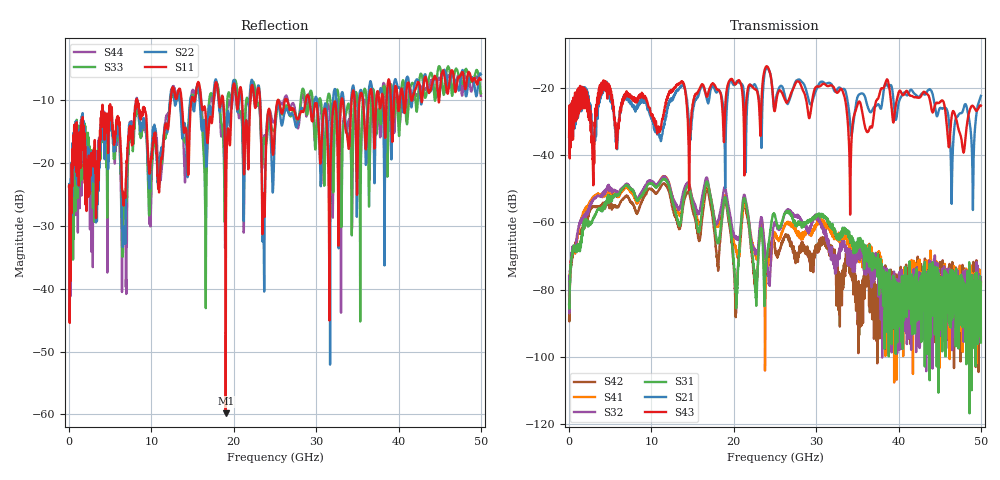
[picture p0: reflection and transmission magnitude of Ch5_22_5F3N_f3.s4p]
!Agilent Technologies,N5247A,US51170199,A.09.90.13
!Agilent N5247A: A.09.90.13
!Date: Wednesday, December 09, 2015 09:21:04
!Correction: S11(Full 4 Port(1,2,3,4))
!S12(Full 4 Port(1,2,3,4))
!S13(Full 4 Port(1,2,3,4))
!S14(Full 4 Port(1,2,3,4))
!S21(Full 4 Port(1,2,3,4))
!S22(Full 4 Port(1,2,3,4))
!S23(Full 4 Port(1,2,3,4))
!S24(Full 4 Port(1,2,3,4))
!S31(Full 4 Port(1,2,3,4))
!S32(Full 4 Port(1,2,3,4))
!S33(Full 4 Port(1,2,3,4))
!S34(Full 4 Port(1,2,3,4))
!S41(Full 4 Port(1,2,3,4))
!S42(Full 4 Port(1,2,3,4))
!S43(Full 4 Port(1,2,3,4))
!S44(Full 4 Port(1,2,3,4))
!S4P File: Measurements: <S11,S12,S13,S14>,
!<S21,S22,S23,S24>,
!<S31,S32,S33,S34>,
!<S41,S42,S43,S44>:
# Hz S  dB  R 50
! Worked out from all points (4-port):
!   3201 points, 10 MHz to 50 GHz, reference 50 ohm
!   strongest paths, dB at 10 MHz, 12.51 GHz, 25 GHz, 37.5 GHz, 50 GHz:
!     S43: -34.5, -21.0, -26.5, -23.2, -25.2
!     S21: -34.5, -23.5, -25.7, -24.8, -22.3
!     S31: -84.5, -53.3, -58.1, -71.7, -95.8
!     S32: -76.1, -52.1, -60.0, -73.0, -76.3
!     S41: -81.5, -52.0, -63.0, -71.4, -77.5
!     S42: -88.9, -55.1, -67.4, -82.6, -77.9
!   lowest |S11| = -59.8 dB at 19.02 GHz (marker M1), VSWR 1.00, Z = 50.1 - j0.0873 ohm
!   |S11| at or under -10 dB: start of sweep to 8.216 GHz; 8.248 GHz to 12.34 GHz (4.093 GHz wide, 39.8 % of centre); 29.18 GHz to 33.06 GHz (3.889 GHz wide, 12.5 % of centre)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
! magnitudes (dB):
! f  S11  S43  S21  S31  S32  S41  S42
! 10 MHz  -23.8  -34.5  -34.5  -84.5  -76.1  -81.5  -88.9
! 3.337 GHz  -20.1  -25.7  -27.1  -56.7  -52.3  -51.6  -55.3
! 19.02 GHz  -59.8  -23.3  -34.8  -53.0  -50.2  -52.3  -53.6
! 20.27 GHz  -9.5  -18.8  -18.4  -81.9  -64.1  -68.2  -87.1
! 21.3 GHz  -19.8  -45.8  -24.6  -52.8  -51.8  -54.0  -54.6
! 22.65 GHz  -11.1  -20.3  -19.3  -78.3  -68.3  -69.8  -79.0
! 50 GHz  -6.7  -25.2  -22.3  -95.8  -76.3  -77.5  -77.9
